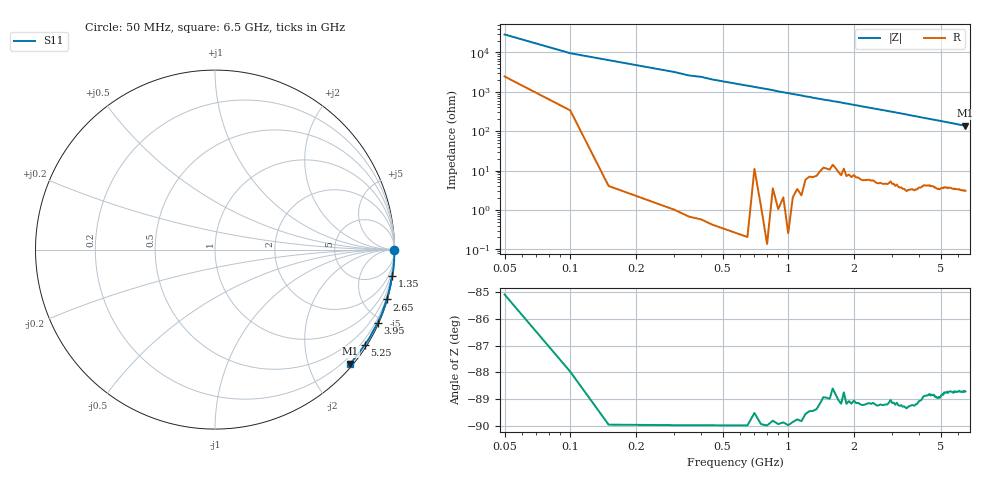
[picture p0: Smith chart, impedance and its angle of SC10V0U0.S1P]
! Infineon Technologies  Discrete & RF Semiconductors
! BAR63-02L
! Si PIN Diode in TSLP-2
! VR = 10 V
! S-Parameters:  March  2002
# GHz  S  MA  R  50
!  f  S11
! GHz  MAG  ANG
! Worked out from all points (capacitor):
!   130 points, 50 MHz to 6.5 GHz, reference 50 ohm
!   read as one part to ground: C = 167 fF near 50 MHz
!   lowest |Z| = 137 ohm at 6.5 GHz (marker M1)
!   S11 on the Smith chart (normalised r, x): 50 MHz: open; 1.35 GHz: 0, -14; 2.65 GHz: 0.10, -7.03; 3.95 GHz: 0.07, -4.64; 5.25 GHz: 0.07, -3.44; 6.5 GHz: 0.06, -2.74
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0.05  0.9997 -0.2
0.35  1 -2.2
0.4  1 -2.4
0.45  1 -2.8
0.85  0.9997 -5.2
0.9  0.9999 -5.6
1.35  0.9984 -8.4
1.55  0.9971 -9.5
1.6  0.9958 -9.9
1.7  0.997 -10.4
1.8  0.9958 -11.1
1.9  0.9968 -11.6
1.95  0.997 -12.0
2  0.9965 -12.2
2.05  0.9968 -12.6
2.1  0.9967 -12.8
2.15  0.9969 -13.2
2.5  0.9963 -15.3
2.65  0.9961 -16.2
3.3  0.9954 -20.2
3.5  0.9959 -21.4
3.95  0.9937 -24.3
4.1  0.9927 -25.3
4.35  0.9912 -26.7
4.9  0.9906 -30.2
5.25  0.9885 -32.4
5.7  0.9877 -35.1
6.5  0.9856 -40.1
